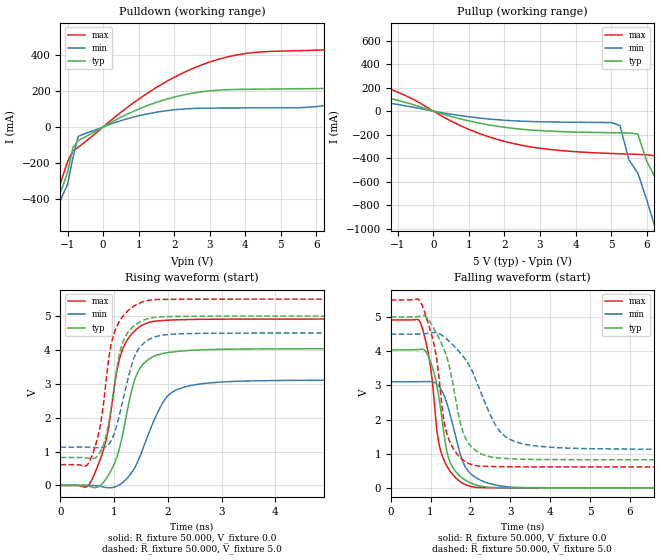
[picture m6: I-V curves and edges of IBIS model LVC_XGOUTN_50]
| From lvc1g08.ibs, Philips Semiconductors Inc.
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|   Model LVC_XGOUTN_50
[Model]   LVC_XGOUTN_50
Model_type   Output
Polarity   Non-Inverting
Vmeas =  2.5V
Cref  =  50.0pF
Rref  =  0.5k
Vref  =  0.0V
C_comp   3.26pF   2.07pF   4.36pF
[Model Spec]
| Note: The input and output voltage ratings may be exceeded if the input and
|   output current ratings are observed (please refer to the data sheet)
|   Subparameter   typ   min   max
| Timing Thresholds
Vmeas   2.5   2.25   2.75
|Ambient temperature:   25   85   -40
[Temperature Range]   50   105   -10
[Voltage Range]   5.0V   4.5V   5.5V
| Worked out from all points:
|   slope of the pulldown table from 0 to 0.75 V, typ, clamps not added: 9.74 ohm
|   slope of the pullup table from 0 to 0.75 V, typ, clamps not added: 11.5 ohm
|   rising waveform, R_fixture 50.000, V_fixture 0.0: 20-80 % time 364ps typ, 508ps min, 352ps max; typ from 0 V to 4.04 V
|   rising waveform, R_fixture 50.000, V_fixture 5.0: 20-80 % time 271ps typ, 332ps min, 289ps max; typ from 0.823 V to 5 V
|   falling waveform, R_fixture 50.000, V_fixture 0.0: 20-80 % time 358ps typ, 462ps min, 338ps max; typ from 4.04 V to 0 V
|   falling waveform, R_fixture 50.000, V_fixture 5.0: 20-80 % time 509ps typ, 817ps min, 393ps max; typ from 5 V to 0.823 V
|Process Range   nominal   slow   fast
[Pulldown]
| voltage   I(typ)   I(min)   I(max)
-5.5V     -4.563A    -4.594A    -4.526A
-1.6V     -693.4mA   -732.2mA   -647.2mA
-1.45V    -551mA     -590.1mA   -504.6mA
-1.3V     -415mA     -454.6mA   -369mA
-1V       -251.4mA   -318mA     -191.1mA
-850mV    -114.6mA   -169.1mA   -132.4mA
-700mV    -75.07mA   -52.23mA   -112.3mA
1.25V     118.3mA    72.36mA    187mA
3V        199.6mA    103.9mA    358.9mA
6.5V      219.2mA    124.2mA    428.1mA
8.5V      324.6mA    195.7mA    566mA
11V       504.2mA    312.6mA    850.5mA
[Pullup]
| voltage   I(typ)   I(min)   I(max)
-6.5V     443.9mA    295.5mA    709.4mA
-2.6V     214.2mA    136.3mA    356.2mA
1.75V     -126.6mA   -72.01mA   -236.6mA
5V        -184mA     -97.72mA   -360.5mA
5.25V     -185.2mA   -121.8mA   -363.2mA
5.5V      -186.8mA   -414.1mA   -365.7mA
5.75V     -193.4mA   -525.3mA   -368mA
6.25V     -569.8mA   -1.001A    -380.6mA
6.75V     -1.057A    -1.508A    -690.7mA
7V        -1.315A    -1.764A    -933.4mA
7.25V     -1.575A    -2.021A    -1.195A
11V       -5.528A    -5.908A    -5.261A
[Ramp]
| variable   typ   min   max
dV/dt_r   2.423V/363.669ps   1.862V/507.696ps   2.948V/351.848ps
dV/dt_f   2.506V/509.027ps   2.022V/816.624ps   2.932V/393.261ps
R_load = 50.000
[Rising Waveform]
R_fixture   = 50.000
V_fixture   = 0.0
V_fixture_min = 0.0
V_fixture_max = 0.0
| time   V(typ)   V(min)   V(max)
0s        266.9pV    3.273nV    21.63pV
500ps     -14.38mV   2.147mV    -34.66mV
850ps     193mV      -64.01mV   1.33V
1.05ns    824.3mV    -22.83mV   3.381V
1.15ns    1.441V     74.18mV    3.985V
1.4ns     3.195V     569mV      4.591V
1.65ns    3.731V     1.563V     4.813V
2ns       3.92V      2.645V     4.878V
2.65ns    4.003V     3.004V     4.904V
9.75ns    4.038V     3.104V     4.913V
[Rising Waveform]
R_fixture   = 50.000
V_fixture   = 5.0
V_fixture_min = 4.5
V_fixture_max = 5.5
| time   V(typ)   V(min)   V(max)
0s        823mV      1.13V      612.8mV
500ps     807.7mV    1.131V     603.6mV
750ps     1.008V     1.11V      1.83V
900ps     1.843V     1.212V     3.769V
1ns       2.92V      1.516V     4.495V
1.2ns     4.372V     2.767V     5.066V
1.35ns    4.685V     3.68V      5.275V
1.55ns    4.881V     4.196V     5.431V
2.45ns    4.993V     4.484V     5.497V
9.75ns    5V         4.5V       5.5V
[Falling Waveform]
R_fixture   = 50.000
V_fixture   = 0.0
V_fixture_min = 0.0
V_fixture_max = 0.0
| time   V(typ)   V(min)   V(max)
0s        4.038V     3.104V     4.913V
750ps     4.054V     3.108V     4.824V
1ns       3.693V     3.11V      3.556V
1.15ns    3.059V     3.048V     1.783V
1.25ns    2.337V     2.911V     1.096V
1.45ns    881.8mV    2.323V     562.4mV
1.75ns    333.2mV    971.6mV    177.6mV
1.9ns     208.6mV    560.7mV    81.53mV
3ns       3.757mV    23.16mV    824.7uV
9.75ns    -11.19uV   -76.02uV   -129.2nV
[Falling Waveform]
R_fixture   = 50.000
V_fixture   = 5.0
V_fixture_min = 4.5
V_fixture_max = 5.5
| time   V(typ)   V(min)   V(max)
0s        5V         4.5V       5.5V
750ps     5.028V     4.504V     5.444V
1.1ns     4.628V     4.546V     4.131V
1.3ns     4.163V     4.455V     2.263V
1.4ns     3.863V     4.361V     1.623V
1.75ns    1.888V     3.944V     883.5mV
1.95ns    1.31V      3.631V     717.8mV
2.65ns    880.1mV    1.802V     621.1mV
3.2ns     842.9mV    1.322V     615.2mV
9.75ns    823.1mV    1.131V     612.8mV
